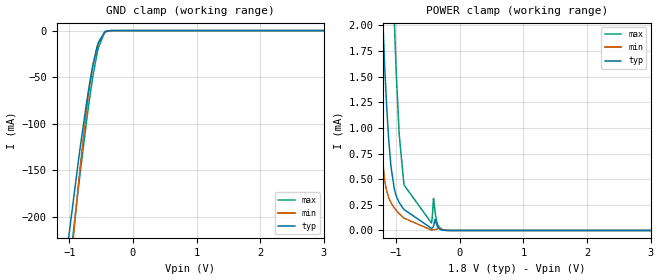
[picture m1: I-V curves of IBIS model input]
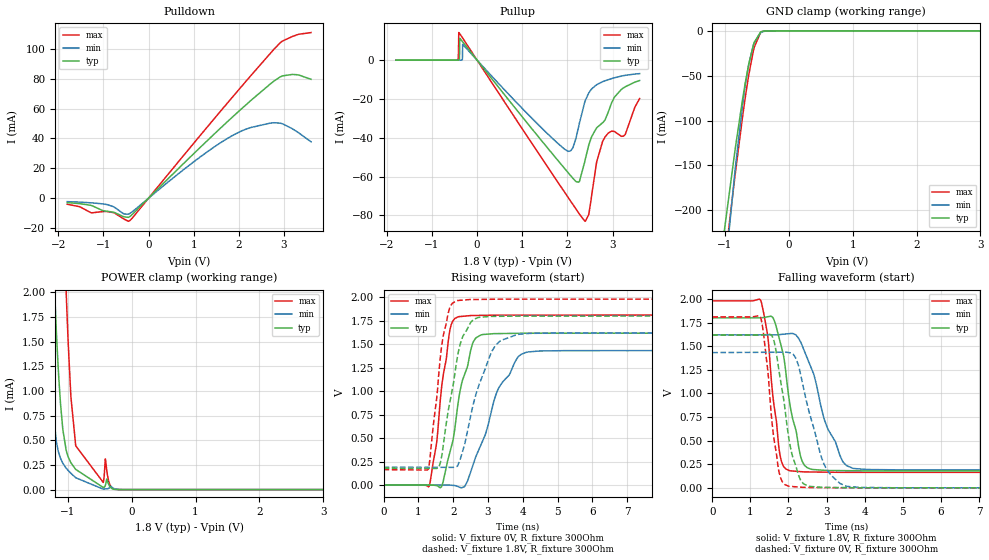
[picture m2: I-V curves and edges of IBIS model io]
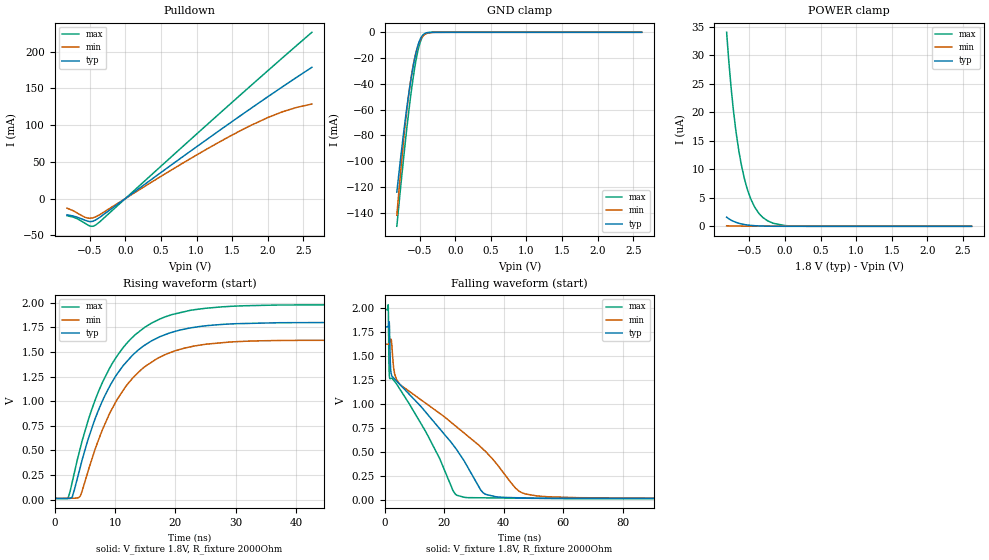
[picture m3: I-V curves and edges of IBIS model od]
|Texas Instruments Incorporated
|TAS2562 6W Boosted Class-D Audio Amplifier with IV-sense
[IBIS Ver]   4.1
[File name]   tas2562.ibs
[Date]   10/10/2018
[File Rev]   1.0
[Source]
| Texas Instruments Incorporated.
| Analog-eLab Design Center, HPA
| 12500 TI Blvd
| Dallas, TX -75243
[Notes]   Revision History:
| Rev 1.0: 10/10/2018
| - Initial version of the model
| - Model generated from simulations in SPECTRE
| - Warnings regarding combined Non-monotonicity of various models
|   have been reviewed and considered minor and can be ignored.
| - C_comp although listed in numerical order of value are
|   obtained from varying PVT conditions. For PVT conditions for
|   each specific value refer the buffer description under
|   respective [Model]. IBIS model user is responsible for using
|   appropriate C_comp to simulate for Signal Integrity.
| - Use "irqz_intpu" model, when internal pullup is used and use
|   "irqz_extpu" model, when external optional pullup is used on IRQZ pin.
[Disclaimer]
| This model is designed as an aid for customers of Texas Instruments.
| TI and its licensors and suppliers make no warranties, either expressed
| or implied, with respect to this  model, including the warranties of
| merchantability or fitness for a particular purpose. The model is
| provided solely on an "as is" basis. The entire risk as to its quality
| and performance is with the customer.
| This model is subject to change without notice. Texas Instruments
| Incorporated is not responsible for updating this model.
[Copyright]
(C) Copyright 2018 Texas Instruments Incorporated.All rights reserved.
|  Component TAS2562YFF 36-pin WCSP (DSBGA) - YFF package
|  Part # TAS2562YFF
[Component]   TAS2562YFF
[Manufacturer]  TI
[Package]   |36 WCSP (DSBGA)- YFF package
|   typ   min   max
R_pkg   0.05   0.04   0.06
L_pkg   1.0nH   0.8nH   1.2nH
C_pkg   0.2pF   0.16pF   0.24pF
[Pin]  signal_name model_name   R_pin   L_pin   C_pin
A1   SDZ   input   NA   NA   NA
A2   SBCLK   io   NA   NA   NA
A3   FSYNC   input   NA   NA   NA
A4   SCL   od   NA   NA   NA
A5   SDA   od   NA   NA   NA
A6   DREG   nc   NA   NA   NA
B1   SDOUT   io   NA   NA   NA
B2   SDIN   io   NA   NA   NA
B3   AD1   input   NA   NA   NA
B4   AD0   input   NA   NA   NA
B5   IRQZ   irqz   NA   NA   NA
B6   VDD   power   NA   NA   NA
C1   VBAT   power   NA   NA   NA
C2   VBAT   power   NA   NA   NA
C3   VSNS_N   nc   NA   NA   NA
C4   GREG   nc   NA   NA   NA
C5   VSNS_P   nc   NA   NA   NA
C6   GPIO   io   NA   NA   NA
D1   BGND   gnd   NA   NA   NA
D2   BGND   gnd   NA   NA   NA
D3   BGND   gnd   NA   NA   NA
D4   GND   gnd   NA   NA   NA
D5   PGND   gnd   NA   NA   NA
D6   PGND   gnd   NA   NA   NA
E1   SW   power   NA   NA   NA
E2   SW   power   NA   NA   NA
E3   SW   power   NA   NA   NA
E4   GND   gnd   NA   NA   NA
E5   OUT_P   nc   NA   NA   NA
E6   OUT_N   nc   NA   NA   NA
F1   VBST   power   NA   NA   NA
F2   VBST   power   NA   NA   NA
F3   VBST   power   NA   NA   NA
F4   PVDD   power   NA   NA   NA
F5   PVDD   power   NA   NA   NA
F6   PVDD   power   NA   NA   NA
|   Model Selectors
[Model Selector] irqz
irqz_intpu   1.8V   digital Output   |Internal Pullup
irqz_extpu   1.8V   digital Open-drain   |External Pullup
| Models and submodels in the file (5): input (Input), io (I/O), od (I/O_open_drain), irqz_intpu (3-state), irqz_extpu (Open_drain)
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|   input Model
[Model]   input
Model_type   Input
Vinl = 0.63
Vinh = 1.17
|   typ   min   max
C_comp   2.003pF   1.966pF   2.088pF
[Model spec]
|subparameter
Vinl   0.63   0.567   0.693
Vinh   1.17   1.053   1.287
| Where Nom  PVT is Nominal Process, 1.8V, 25C
|   Fast PVT is Strong Process,  1.98V, -40C
|   Slow PVT is Weak Process,   1.62V, 150C
[Voltage Range]   1.8   1.62   1.98
|Junction Temperature
[Temperature Range]   25   150   -40
[Power Clamp Reference]   1.8   1.62   1.98
[GND Clamp Reference]   0   0   0
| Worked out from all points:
|   GND clamp passes 1 mA (typ) near -0.43 V on its own axis
|   POWER clamp passes 1 mA (typ) near -1.13 V on its own axis
[GND Clamp]
|   Voltage   I(typ)   I(min)   I(max)
-1.8V     -830.2mA   -917.2mA   -810.3mA
-1.017V   -226mA     -280.9mA   -265mA
-849.6mV  -136.2mA   -160.2mA   -164.9mA
-725.4mV  -76.2mA    -82.49mA   -95.68mA
-676.8mV  -55.51mA   -57.51mA   -71.17mA
-628.2mV  -37.22mA   -36.99mA   -48.97mA
-558mV    -16.53mA   -16.23mA   -22.83mA
-541.8mV  -12.94mA   -12.9mA    -18.1mA
-439.2mV  -1.277mA   -1.972mA   -1.711mA
-385.2mV  -225.2uA   -567.9uA   -219.6uA
-261mV    -2.196uA   -22.38uA   -650.9nA
3.6V      0A         0A         0A
[POWER Clamp]
|   Voltage   I(typ)   I(min)   I(max)
-1.8V     15.69mA    11.82mA    24.27mA
-1.352V   4.592mA    2.132mA    9.4mA
-1.249V   2.667mA    900.4uA    6.926mA
-1.152V   1.249mA    396.7uA    4.653mA
-1.082V   632.3uA    271.2uA    3.097mA
-1.022V   390.1uA    214.6uA    1.943mA
-952.2mV  272.5uA    165.5uA    941.7uA
-876.6mV  204.9uA    120.4uA    444.5uA
-444.6mV  21.3uA     4.377uA    72.73uA
-412.2mV  43.5uA     7.407uA    311.6uA
-261mV    1.982uA    6.997uA    3.319uA
3.6V      0A         0A         0A
|   i0 Model
[Model]   io
Model_type   I/O
Polarity   Non-Inverting
Enable   Active-Low
Vinl = 0.63
Vinh = 1.17
Vmeas = 0.9
Vref = 0
Cref = 2pF
Rref = 100000
|   typ   min   max
C_comp   2.003pF   1.966pF   2.088pF
[Model spec]
|subparameter
Vinl   0.63   0.567   0.693
Vinh   1.17   1.053   1.287
| Where Nom  PVT is Nominal Process, 1.8V, 25C
|   Fast PVT is Strong Process,  1.98V, -40C
|   Slow PVT is Weak Process,   1.62V, 150C
[Voltage Range]   1.8   1.62   1.98
|Junction Temperature
[Temperature Range]   25   150   -40
[Pullup Reference]   1.8   1.62   1.98
[Pulldown Reference]   0   0   0
[Power Clamp Reference]   1.8   1.62   1.98
[GND Clamp Reference]   0   0   0
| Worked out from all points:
|   slope of the pulldown table from 0 to 0.27 V, typ, clamps not added: 33.2 ohm
|   slope of the pullup table from 0 to 0.27 V, typ, clamps not added: 33.9 ohm
|   GND clamp passes 1 mA (typ) near -0.43 V on its own axis
|   POWER clamp passes 1 mA (typ) near -1.13 V on its own axis
|   falling waveform, V_fixture 1.8V, R_fixture 300Ohm: 20-80 % time 416ps typ, 711ps min, 272ps max; typ from 1.8 V to 0.179 V
|   rising waveform, V_fixture 0V, R_fixture 300Ohm: 20-80 % time 541ps typ, 907ps min, 349ps max; typ from 0 V to 1.62 V
|   rising waveform, V_fixture 1.8V, R_fixture 300Ohm: 20-80 % time 441ps typ, 657ps min, 333ps max; typ from 0.179 V to 1.8 V
|   falling waveform, V_fixture 0V, R_fixture 300Ohm: 20-80 % time 384ps typ, 551ps min, 287ps max; typ from 1.62 V to 0 V
[Pulldown]
|   Voltage   I(typ)   I(min)   I(max)
-1.8V     -2.957mA   -2.3mA     -4.034mA
-1.525V   -3.634mA   -2.61mA    -5.679mA
-1.26V    -4.892mA   -3.1mA     -9.788mA
-925.2mV  -8.723mA   -4.215mA   -8.896mA
-547.2mV  -12.42mA   -10.54mA   -13.89mA
-412.2mV  -12.21mA   -10.16mA   -14.9mA
1.219V    36.12mA    29.23mA    44.65mA
2.158V    62.44mA    46.19mA    78.22mA
2.687V    76.17mA    50.19mA    96.55mA
2.957V    81.7mA     49.87mA    104.9mA
3.276V    82.66mA    44.75mA    109.2mA
3.6V      79.58mA    37.74mA    110.8mA
[GND Clamp]
|   Voltage   I(typ)   I(min)   I(max)
-1.8V     -830.2mA   -917.2mA   -810.3mA
-1.017V   -226mA     -280.9mA   -265mA
-849.6mV  -136.2mA   -160.2mA   -164.9mA
-725.4mV  -76.2mA    -82.49mA   -95.68mA
-676.8mV  -55.51mA   -57.51mA   -71.17mA
-628.2mV  -37.22mA   -36.99mA   -48.97mA
-558mV    -16.53mA   -16.23mA   -22.83mA
-541.8mV  -12.94mA   -12.9mA    -18.1mA
-439.2mV  -1.277mA   -1.972mA   -1.711mA
-385.2mV  -225.2uA   -567.9uA   -219.6uA
-261mV    -2.196uA   -22.37uA   -650.9nA
3.6V      0A         0A         0A
[Pullup]
|   Voltage   I(typ)   I(min)   I(max)
-1.8V     1.307nA    3.762nA    3.133nA
-444.6mV  644.7nA    9.633nA    21.14uA
-417.6mV  10.83uA    113.9nA    482.6uA
-406.8mV  33.57uA    111.3nA    14.24mA
-385.2mV  11.32mA    357.5nA    13.58mA
-320.4mV  9.469mA    8.197mA    11.39mA
2.002V    -57.57mA   -46.79mA   -70.24mA
2.25V     -62.85mA   -34.12mA   -78.78mA
2.396V    -51.09mA   -20.79mA   -83.03mA
2.779V    -32.25mA   -11.09mA   -41.92mA
3.276V    -13.77mA   -7.821mA   -38.42mA
3.6V      -10.46mA   -6.92mA    -19.73mA
[POWER Clamp]
|   Voltage   I(typ)   I(min)   I(max)
-1.8V     15.69mA    11.82mA    24.27mA
-1.352V   4.592mA    2.132mA    9.4mA
-1.249V   2.668mA    900.4uA    6.926mA
-1.152V   1.249mA    396.7uA    4.653mA
-1.082V   632.3uA    271.2uA    3.097mA
-1.022V   390.1uA    214.6uA    1.943mA
-952.2mV  272.5uA    165.5uA    941.7uA
-876.6mV  204.9uA    120.4uA    444.5uA
-444.6mV  21.3uA     4.377uA    72.73uA
-412.2mV  43.5uA     7.407uA    311.6uA
-261mV    1.982uA    6.997uA    3.298uA
3.6V      0A         0A         0A
[Ramp]
R_load = 300
|   typ   min   max
dV/dt_r   0.970304/5.44182e-10   0.85939/9.22655e-10   1.08617/3.49721e-10
dV/dt_f   0.972502/4.13666e-10   0.858487/7.13239e-10   1.08978/2.70627e-10
[Falling Waveform]
V_fixture = 1.8V
V_fixture_min = 1.62V
V_fixture_max = 1.98V
R_fixture = 300Ohm
C_fixture = 0F
|   Time   V(typ)   V(min)   V(max)
0s        1.8V       1.62V      1.98V
1.269ns   1.8V       1.62V      1.988V
1.461ns   1.812V     1.62V      1.59V
1.581ns   1.807V     1.62V      1.007V
1.772ns   1.559V     1.623V     359.2mV
2.021ns   929.8mV    1.633V     182.8mV
2.424ns   236.8mV    1.441V     168.9mV
3.016ns   184.3mV    639.9mV    166.1mV
3.686ns   181.4mV    207.5mV    164.3mV
16.67ns   179.2mV    189.2mV    163.7mV
[Rising Waveform]
V_fixture = 0V
V_fixture_min = 0V
V_fixture_max = 0V
R_fixture = 300Ohm
C_fixture = 0F
|   Time   V(typ)   V(min)   V(max)
0s        433nV      -1.36uV    1.007uV
1.308ns   -67.01uV   -73.62uV   -12.78mV
1.525ns   -6.579mV   -85.61uV   457mV
1.666ns   -16.36mV   -93.39uV   1.04V
1.914ns   363.3mV    -1.182mV   1.669V
2.137ns   863.3mV    -16.65mV   1.791V
2.647ns   1.566V     298.8mV    1.806V
3.295ns   1.613V     1.024V     1.81V
4.091ns   1.616V     1.412V     1.81V
16.67ns   1.617V     1.432V     1.81V
[Rising Waveform]
V_fixture = 1.8V
V_fixture_min = 1.62V
V_fixture_max = 1.98V
R_fixture = 300Ohm
C_fixture = 0F
|   Time   V(typ)   V(min)   V(max)
0s        179.2mV    189.2mV    163.7mV
1.28ns    176.9mV    188.4mV    167.5mV
1.585ns   185.7mV    188.2mV    1.184V
1.698ns   380.9mV    188.1mV    1.558V
1.892ns   861.4mV    188mV      1.879V
2.096ns   1.309V     195.9mV    1.962V
2.504ns   1.732V     738.7mV    1.976V
3.081ns   1.796V     1.4V       1.978V
3.825ns   1.799V     1.601V     1.98V
16.67ns   1.8V       1.62V      1.98V
[Falling Waveform]
|Gnd
V_fixture = 0V
V_fixture_min = 0V
V_fixture_max = 0V
R_fixture = 300Ohm
C_fixture = 0F
|   Time   V(typ)   V(min)   V(max)
0s        1.617V     1.432V     1.81V
1.262ns   1.617V     1.435V     1.811V
1.449ns   1.624V     1.435V     1.268V
1.624ns   1.549V     1.436V     505.2mV
1.783ns   1.157V     1.436V     115.6mV
1.994ns   562.2mV    1.433V     18.68mV
2.394ns   42.83mV    1.059V     5.177mV
2.931ns   5.209mV    253.2mV    2.738mV
3.519ns   2.625mV    17.64mV    561.1uV
16.67ns   -371.2nV   -1.224uV   996.7nV
|   od Model
[Model]   od
Model_type   I/O_open_drain
Polarity   Non-Inverting
Enable   Active-Low
Vinl = 0.54
Vinh = 1.26
Vmeas = 0.9
Vref = 1.8
Cref = 2pF
Rref = 2000
|   typ   min   max
C_comp   1.948pF   1.939pF   1.994pF
[Model spec]
|subparameter
Vinl   0.54   0.486   0.594
Vinh   1.26   1.134   1.386
| Where Nom  PVT is Nominal Process, 1.8V, 25C
|   Fast PVT is Strong Process,  1.98V, -40C
|   Slow PVT is Weak Process,   1.62V, 150C
[Voltage Range]   1.8   1.62   1.98
|Junction Temperature
[Temperature Range]   25   150   -40
[Pullup Reference]   1.8   1.62   1.98
[Pulldown Reference]   0   0   0
[Power Clamp Reference]   1.8   1.62   1.98
[GND Clamp Reference]   0   0   0
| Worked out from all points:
|   slope of the pulldown table from 0 to 0.27 V, typ, clamps not added: 14.1 ohm
|   GND clamp passes 1 mA (typ) near -0.43 V on its own axis
|   falling waveform, V_fixture 1.8V, R_fixture 2000Ohm: 20-80 % time 25.4ns typ, 35.1ns min, 17.4ns max; typ from 1.8 V to 0.013 V
|   rising waveform, V_fixture 1.8V, R_fixture 2000Ohm: 20-80 % time 8.14ns typ, 8.23ns min, 8.18ns max; typ from 0.013 V to 1.8 V
[Pulldown]
|   Voltage   I(typ)   I(min)   I(max)
-820mV    -22.14mA   -13.11mA   -23.32mA
-692.7mV  -24.89mA   -18.8mA    -26.79mA
-568.9mV  -29.43mA   -25.45mA   -33.52mA
-472.6mV  -31.22mA   -26.59mA   -37.77mA
-417.5mV  -29.18mA   -24.86mA   -36.06mA
814mV     57.45mA    48.59mA    71.47mA
1.591V    111mA      91.06mA    138.9mA
2.004V    138.7mA    110.3mA    174.2mA
2.211V    152.3mA    118.2mA    191.7mA
2.407V    165mA      124mA      208.3mA
2.62V     178.5mA    128.6mA    226.2mA
[GND Clamp]
|   Voltage   I(typ)   I(min)   I(max)
-820mV    -123.9mA   -141.9mA   -150.4mA
-765mV    -96.74mA   -107mA     -119.3mA
-713.4mV  -72.95mA   -77.5mA    -91.56mA
-672.1mV  -55.44mA   -56.84mA   -70.82mA
-623.9mV  -37.25mA   -36.82mA   -48.8mA
-575.8mV  -22.16mA   -21.63mA   -29.95mA
-524.2mV  -10.31mA   -10.61mA   -14.49mA
-482.9mV  -4.466mA   -5.26mA    -6.382mA
-431.3mV  -1.128mA   -1.849mA   -1.462mA
-390mV    -299.2uA   -716.9uA   -303uA
-297.1mV  -10.05uA   -67.24uA   -4.271uA
2.62V     0A         0A         0A
[POWER Clamp]
|   Voltage   I(typ)   I(min)   I(max)
-820mV    1.599uA    92.71nA    34.07uA
-792.5mV  1.347uA    74.43nA    29.43uA
-727.1mV  894.9nA    54.66nA    20.64uA
-682.4mV  670.4nA    45.24nA    16.08uA
-617mV    432.8nA    35.66nA    11.03uA
-548.2mV  267.2nA    29.35nA    7.314uA
-476mV    156.4nA    25.16nA    4.668uA
-376.2mV  69.94nA    22nA       2.43uA
-307.4mV  37.44nA    20.77nA    1.513uA
-166.4mV  6.224nA    19.34nA    534.3nA
98.48mV   0A         17.8nA     51.98nA
2.62V     0A         0A         0A
[Ramp]
R_load = 2000
|   typ   min   max
dV/dt_r   1.07247/8.12164e-09   0.964105/8.20765e-09   1.18114/8.18063e-09
dV/dt_f   1.07247/2.54587e-08   0.964105/3.5158e-08   1.18114/1.74515e-08
[Falling Waveform]
V_fixture = 1.8V
V_fixture_min = 1.62V
V_fixture_max = 1.98V
R_fixture = 2000Ohm
C_fixture = 0F
|   Time   V(typ)   V(min)   V(max)
0s        1.8V       1.62V      1.98V
1.218ns   1.8V       1.62V      2.031V
1.491ns   1.853V     1.62V      1.381V
1.724ns   1.688V     1.637V     1.263V
2.465ns   1.288V     1.595V     1.266V
5.077ns   1.202V     1.204V     1.154V
26.81ns   400.2mV    692.4mV    25.25mV
33.85ns   56.98mV    504.4mV    20.08mV
50.9ns    16.87mV    41.09mV    14.71mV
250ns     12.54mV    13.11mV    11.15mV
[Rising Waveform]
V_fixture = 1.8V
V_fixture_min = 1.62V
V_fixture_max = 1.98V
R_fixture = 2000Ohm
C_fixture = 0F
|   Time   V(typ)   V(min)   V(max)
0s        12.54mV    13.11mV    11.15mV
2.215ns   12.52mV    14.28mV    15.98mV
2.912ns   30.52mV    14.64mV    183.5mV
4.209ns   326.2mV    35.04mV    518.2mV
5.635ns   632.9mV    311.7mV    824.5mV
7.564ns   955.8mV    656.8mV    1.143V
11.33ns   1.36V      1.108V     1.543V
17.05ns   1.643V     1.435V     1.823V
24.91ns   1.764V     1.577V     1.943V
250ns     1.8V       1.62V      1.98V
